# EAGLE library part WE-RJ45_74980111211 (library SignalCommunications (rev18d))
Order Code 74980111211 Design SMD xBase-T 10/100 Base-T Ports 1x1 Application Standard Tab Position Up LED (Left-Right) YELLOW-GREEN EMI Fingers Yes Details see: http://katalog.we-online.de/en/pbs/WE-LAN_RJ45/74980111211? Updated by Yingchun Shan 2016-08-23 2014 (C) Würth Elektronik
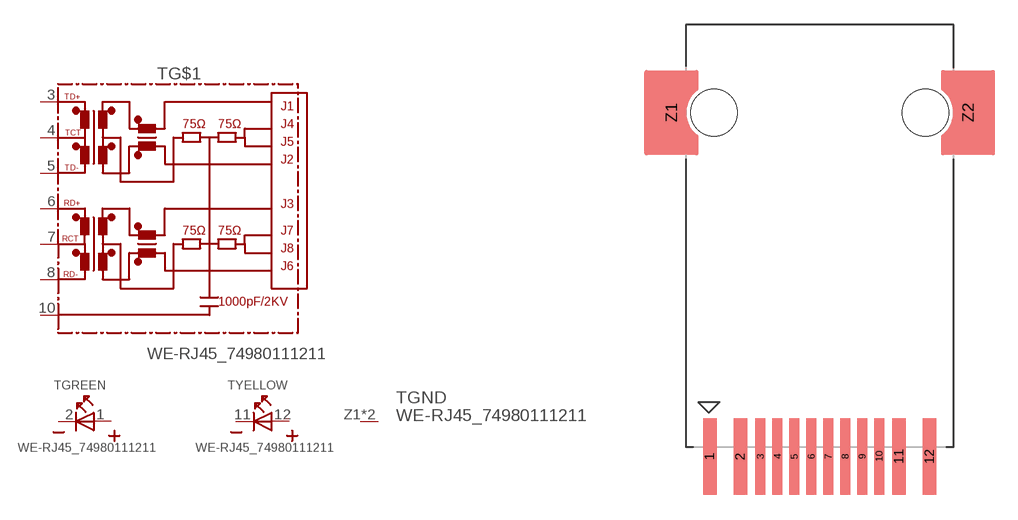
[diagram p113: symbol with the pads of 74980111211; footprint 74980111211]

Designator prefix T; gates G$1=74980111211 GND=GNDPIN GREEN=LED-2PIN YELLOW=LED-2PIN

## WE-RJ45_74980111211 (COMPANY-URL: http://www.we-online.de; CREATED-BY: Christin Zierenner; CREATED-DATE: AUG 2012; DATASHEET-URL: http://katalog.we-online.de/kataloge/eisos/media/pdf/74980111211.pdf; MANUFACTURER: Würth Elektronik eiSos GmbH)  [74980111211]
1  GREEN:A  pas
2  GREEN:K  pas
3  G$1:TD+
4  G$1:TCT
5  G$1:TD-
6  G$1:RD+
7  G$1:RCT
8  G$1:RD-
10  G$1:8
11  YELLOW:K  pas
12  YELLOW:A  pas
Z1  GND:GND  pwr
Z2  GND:GND  pwr

## Footprint 74980111211 (pad centres in mm)
MAX HEIGHT=13.61mm PORTS----1X1 LED --Yes
smd 0.81 x 4.6: 1 -6.61,-20.69; 2 -4.77,-20.69; 11 4.77,-20.69; 12 6.61,-20.69
smd 0.61 x 4.6: 3 -3.57,-20.69; 4 -2.55,-20.69; 5 -1.53,-20.69; 6 -0.51,-20.69; 7 0.51,-20.69; 8 1.53,-20.69; 9 2.55,-20.69; 10 3.57,-20.69
smd 1 x 4.9: Z1 -8.92,0; Z2 8.92,0
hole 2.8 at 6.35,0
hole 2.8 at -6.35,0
